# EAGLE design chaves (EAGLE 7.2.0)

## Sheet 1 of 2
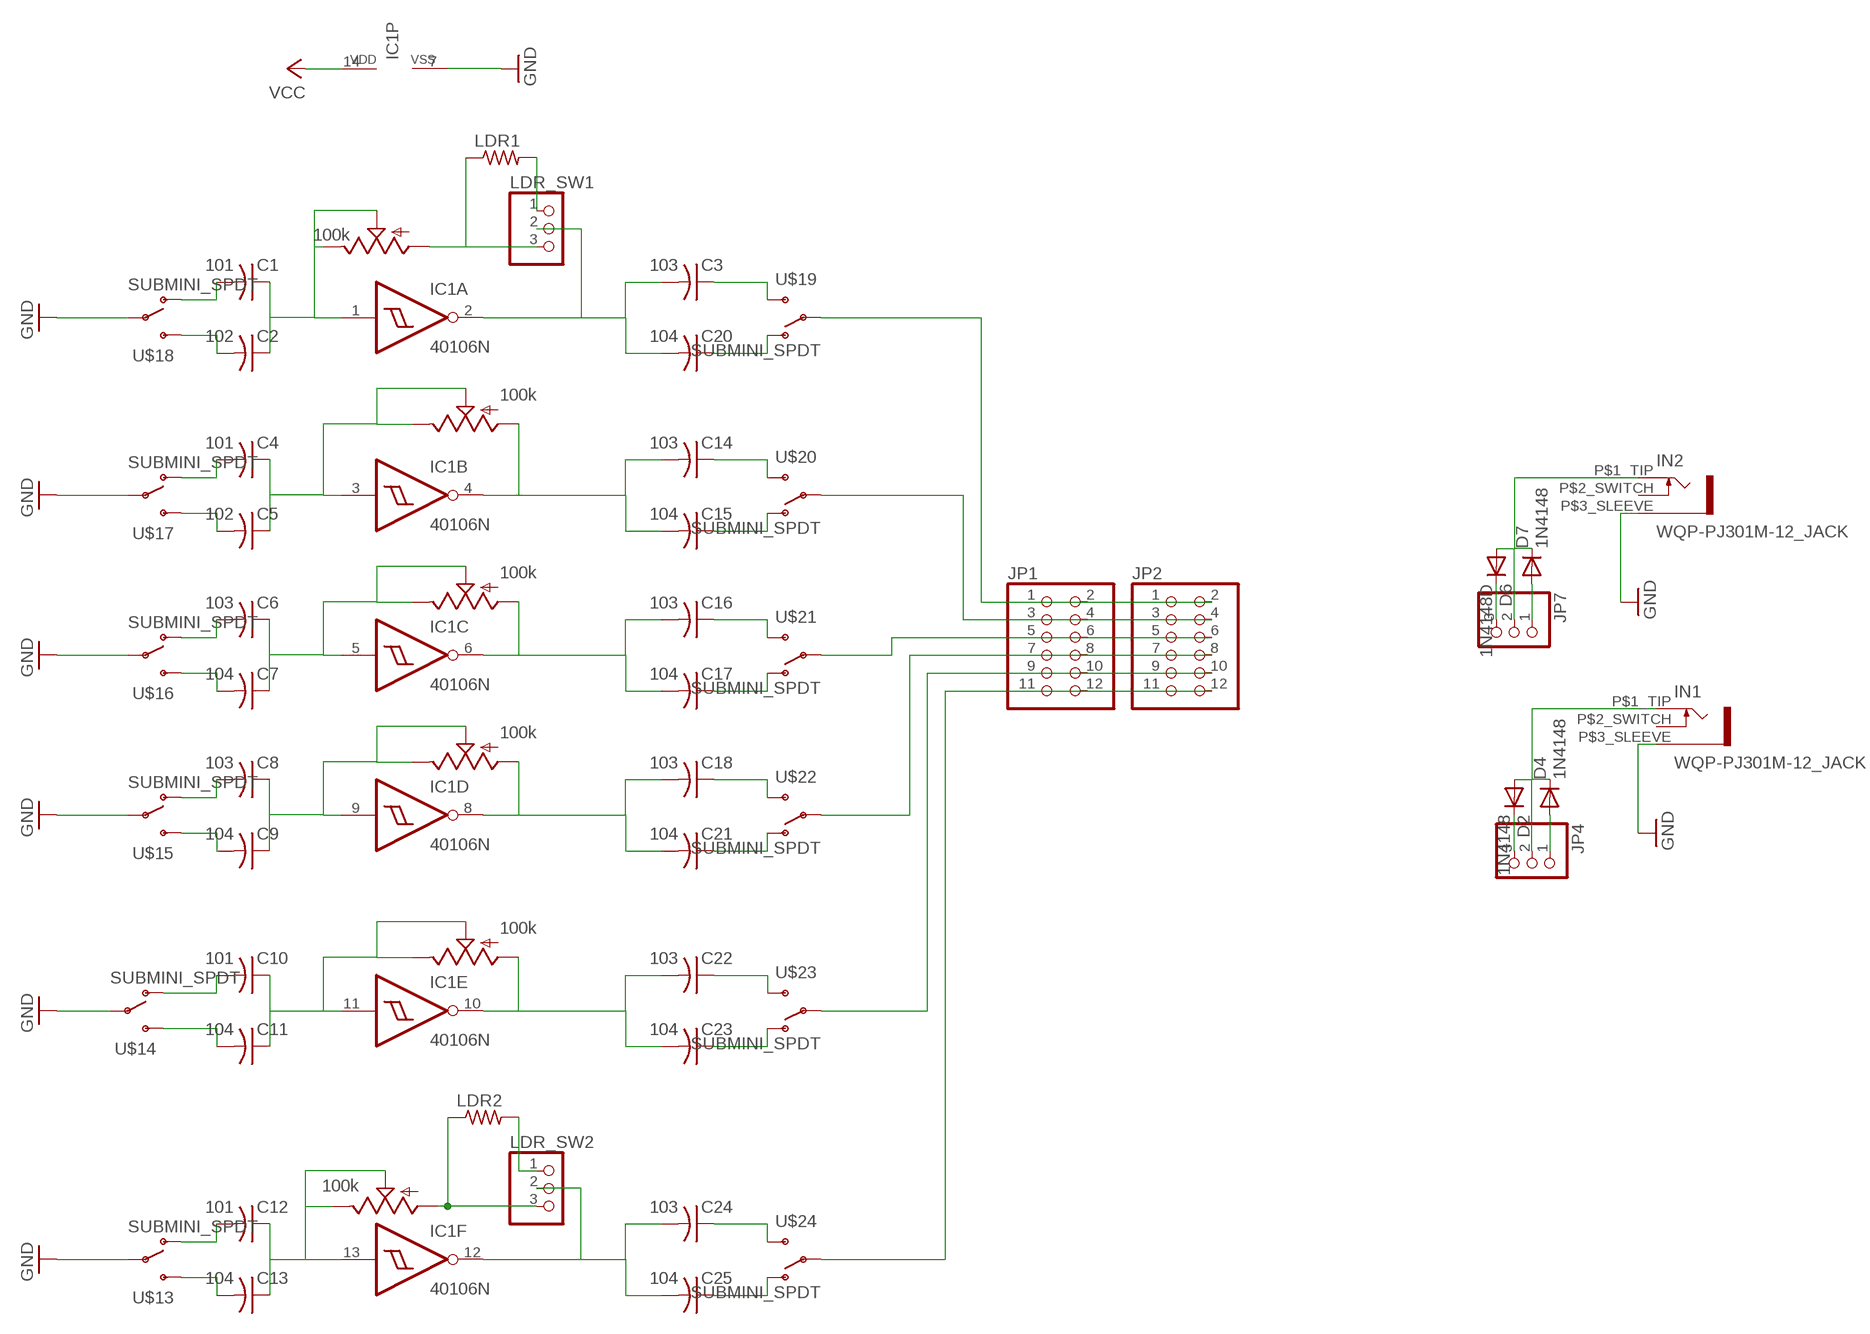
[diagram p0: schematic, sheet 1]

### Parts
C1  101  C-US050-025X075  [C050-025X075]
C2  102  C-US050-025X075  [C050-025X075]
C3  103  C-US050-025X075  [C050-025X075]
C4  101  C-US050-025X075  [C050-025X075]
C5  102  C-US050-025X075  [C050-025X075]
C6  103  C-US050-025X075  [C050-025X075]
C7  104  C-US050-025X075  [C050-025X075]
C8  103  C-US050-025X075  [C050-025X075]
C9  104  C-US050-025X075  [C050-025X075]
C10  101  C-US050-025X075  [C050-025X075]
C11  104  C-US050-025X075  [C050-025X075]
C12  101  C-US050-025X075  [C050-025X075]
C13  104  C-US050-025X075  [C050-025X075]
C14  103  C-US050-025X075  [C050-025X075]
C15  104  C-US050-025X075  [C050-025X075]
C16  103  C-US050-025X075  [C050-025X075]
C17  104  C-US050-025X075  [C050-025X075]
C18  103  C-US050-025X075  [C050-025X075]
C20  104  C-US050-025X075  [C050-025X075]
C21  104  C-US050-025X075  [C050-025X075]
C22  103  C-US050-025X075  [C050-025X075]
C23  104  C-US050-025X075  [C050-025X075]
C24  103  C-US050-025X075  [C050-025X075]
C25  104  C-US050-025X075  [C050-025X075]
D2  1N4148  1N4148DO35-7  [DO35-7]
D4  1N4148  1N4148DO35-7  [DO35-7]
D6  1N4148D  1N4148DO35-7  [DO35-7]
D7  1N4148  1N4148DO35-7  [DO35-7]
IC1  40106N  [DIL14]
IN1  WQP-PJ301M-12_JACK  [WQP-PJ301M-12_JACK]
IN2  WQP-PJ301M-12_JACK  [WQP-PJ301M-12_JACK]
JP1  PINHD-2X6  [2X06]
JP2  PINHD-2X6  [2X06]
JP4  PINHD-1X3CB  [1X03-CLEANBIG]
JP7  PINHD-1X3CB  [1X03-CLEANBIG]
LDR1  R-US_0204/7  [0204/7]
LDR2  R-US_0204/7  [0204/7]
LDR_SW1  PINHD-1X3  [1X03]
LDR_SW2  PINHD-1X3  [1X03]
POT1  100k  POT_USVERTICAL  [ALPS_POT_VERTICAL]
POT2  100k  POT_USVERTICAL  [ALPS_POT_VERTICAL]
POT3  100k  POT_USVERTICAL  [ALPS_POT_VERTICAL]
POT4  100k  POT_USVERTICAL  [ALPS_POT_VERTICAL]
POT5  100k  POT_USVERTICAL  [ALPS_POT_VERTICAL]
POT6  100k  POT_USVERTICAL  [ALPS_POT_VERTICAL]
U$13  SUBMINI_SPDT  [SUBMINI_TOGGLE]
U$14  SUBMINI_SPDT  [SUBMINI_TOGGLE]
U$15  SUBMINI_SPDT  [SUBMINI_TOGGLE]
U$16  SUBMINI_SPDT  [SUBMINI_TOGGLE]
U$17  SUBMINI_SPDT  [SUBMINI_TOGGLE]
U$18  SUBMINI_SPDT  [SUBMINI_TOGGLE]
U$19  SUBMINI_SPDT  [SUBMINI_TOGGLE]
U$20  SUBMINI_SPDT  [SUBMINI_TOGGLE]
U$21  SUBMINI_SPDT  [SUBMINI_TOGGLE]
U$22  SUBMINI_SPDT  [SUBMINI_TOGGLE]
U$23  SUBMINI_SPDT  [SUBMINI_TOGGLE]
U$24  SUBMINI_SPDT  [SUBMINI_TOGGLE]

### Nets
GND: IC1.7(P:VSS) IN1.P$3_SLEEVE IN2.P$3_SLEEVE U$13.COM(COMMON) U$14.COM(COMMON) U$15.COM(COMMON) U$16.COM(COMMON) U$17.COM(COMMON) U$18.COM(COMMON) ; also sheet 2
GND1: C3.2 C20.2 IC1.2(A:O) LDR_SW1.2
GND2: C14.2 C15.2 IC1.4(B:O) POT2.P$3(A)
GND3: C16.2 C17.2 IC1.6(C:O) POT3.P$3(A)
GND4: C18.2 C21.2 IC1.8(D:O) POT4.P$3(A)
GND5: C22.2 C23.2 IC1.10(E:O) POT5.P$3(A)
GND6: C24.2 C25.2 IC1.12(F:O) LDR_SW2.2
N$1: C1.2 U$18.1(O)
N$2: C2.2 U$18.3(S)
N$3: LDR2.2 LDR_SW2.1
N$4: C5.2 U$17.3(S)
N$5: C4.2 U$17.1(O)
N$6: LDR1.2 LDR_SW1.1
N$7: C8.2 U$15.1(O)
N$8: C9.2 U$15.3(S)
N$9: D6.A D7.C IN2.P$1_TIP JP7.2
N$10: C6.2 U$16.1(O)
N$11: C7.2 U$16.3(S)
N$16: C20.1 U$19.1(O)
N$17: C3.1 U$19.3(S)
N$18: JP1.1 JP1.2 JP2.1 JP2.2 U$19.COM(COMMON)
N$19: LDR1.1 LDR_SW1.3 POT1.P$3(A)
N$22: LDR2.1 LDR_SW2.3 POT6.P$3(A)
N$23: D2.A D4.C IN1.P$1_TIP JP4.2
N$24: C15.1 U$20.1(O)
N$26: C14.1 U$20.3(S)
N$27: JP1.3 JP1.4 JP2.3 JP2.4 U$20.COM(COMMON)
N$28: C17.1 U$21.1(O)
N$29: C16.1 U$21.3(S)
N$30: JP1.5 JP1.6 JP2.5 JP2.6 U$21.COM(COMMON)
N$31: C1.1 C2.1 IC1.1(A:I) POT1.P$1(E) POT1.P$2(S)
N$32: C4.1 C5.1 IC1.3(B:I) POT2.P$1(E) POT2.P$2(S)
N$33: C6.1 C7.1 IC1.5(C:I) POT3.P$1(E) POT3.P$2(S)
N$34: C8.1 C9.1 IC1.9(D:I) POT4.P$1(E) POT4.P$2(S)
N$37: C21.1 U$22.1(O)
N$38: C18.1 U$22.3(S)
N$39: JP1.7 JP1.8 JP2.7 JP2.8 U$22.COM(COMMON)
N$40: C23.1 U$23.1(O)
N$41: C22.1 U$23.3(S)
N$42: JP1.9 JP1.10 JP2.9 JP2.10 U$23.COM(COMMON)
N$43: C25.1 U$24.1(O)
N$44: C24.1 U$24.3(S)
N$45: JP1.11 JP1.12 JP2.11 JP2.12 U$24.COM(COMMON)
N$46: C10.2 U$14.1(O)
N$47: C10.1 C11.1 IC1.11(E:I) POT5.P$1(E) POT5.P$2(S)
N$48: C11.2 U$14.3(S)
N$49: C13.2 U$13.3(S)
N$50: C12.2 U$13.1(O)
N$51: C12.1 C13.1 IC1.13(F:I) POT6.P$1(E) POT6.P$2(S)
N$52: D2.C JP4.3
N$53: D4.A JP4.1
N$56: D6.C JP7.3
N$58: D7.A JP7.1
VCC: IC1.14(P:VDD) ; also sheet 2
Unconnected: IN1.P$2_SWITCH IN2.P$2_SWITCH

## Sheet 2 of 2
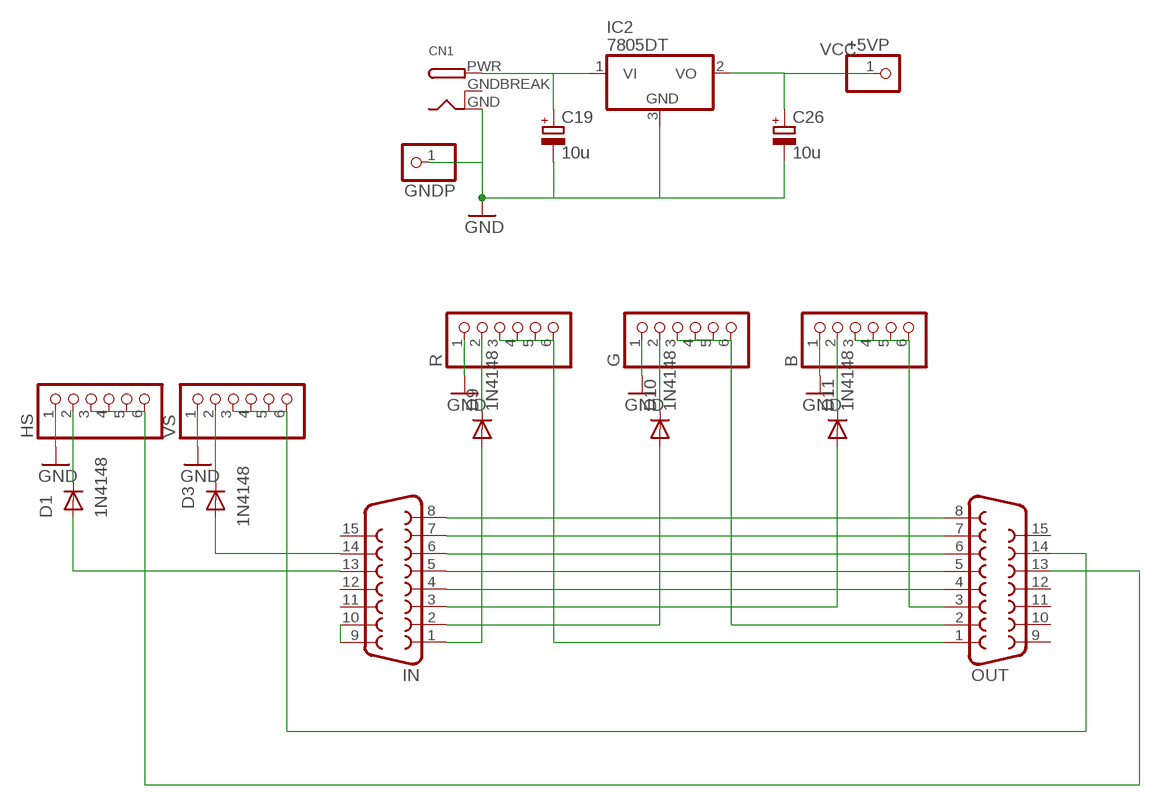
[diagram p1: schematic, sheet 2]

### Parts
+5VP  PINHD-1X1CB  [1X01-CLEANBIG]
B  PINHD-1X6CLEAN  [1X06-CLEAN]
C19  10u  CPOL-EUE2.5-5  [E2,5-5]
C26  10u  CPOL-EUE2.5-5  [E2,5-5]
CN1  DCBARRELPTH  [DCJACK_2MM_PTH]
D1  1N4148  1N4148DO35-7  [DO35-7]
D3  1N4148  1N4148DO35-7  [DO35-7]
D9  1N4148  1N4148DO35-7  [DO35-7]
D10  1N4148  1N4148DO35-7  [DO35-7]
D11  1N4148  1N4148DO35-7  [DO35-7]
G  PINHD-1X6CLEAN  [1X06-CLEAN]
GNDP  PINHD-1X1CB  [1X01-CLEANBIG]
HS  PINHD-1X6CLEAN  [1X06-CLEAN]
IC2  7805DT  [TO252]
IN  F15HDH  [HDF15H]
OUT  F15HDH  [HDF15H]
R  PINHD-1X6CLEAN  [1X06-CLEAN]
VS  PINHD-1X6CLEAN  [1X06-CLEAN]

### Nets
GND: B.1 C19.- C26.- CN1.GND G.1 GNDP.1 HS.1 IC2.3(GND) IN.4 IN.5 IN.6 IN.7 IN.8 IN.9 IN.10 OUT.4 OUT.5 OUT.6 OUT.7 OUT.8 R.1 VS.1 ; also sheet 1
N$12: D9.A IN.1
N$13: D9.C R.2
N$14: OUT.1 R.3 R.4 R.5 R.6
N$15: D10.A IN.2
N$20: D10.C G.2
N$21: G.3 G.4 G.5 G.6 OUT.2
N$25: D11.A IN.3
N$35: B.2 D11.C
N$36: B.3 B.4 B.5 B.6 OUT.3
N$54: OUT.14 VS.3 VS.4 VS.5 VS.6
N$55: HS.3 HS.4 HS.5 HS.6 OUT.13
N$57: C19.+ CN1.PWR IC2.1(VI)
N$60: D1.C HS.2
N$62: D1.A IN.13
N$63: D3.A IN.14
N$64: D3.C VS.2
VCC: +5VP.1 C26.+ IC2.2(VO) ; also sheet 1
Unconnected: IN.11 IN.12 IN.15 OUT.9 OUT.10 OUT.11 OUT.12 OUT.15

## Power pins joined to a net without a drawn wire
GNDBREAK: CN1.GNDBREAK

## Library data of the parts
+5VP GNDP = adafruit:PINHD-1X1: Pin header 1x1 for 0.1" spacing
B G HS R VS = adafruit:PINHD-1X6: PIN HEADER
C1-C18 C20-C25 = adafruit:C-US: CAPACITOR, American symbol
C19 C26 = rcl:CPOL-EU: POLARIZED CAPACITOR, European symbol
CN1 = adafruit:DCBARREL: 2.0mm DC Barrel Jack DCJACK_2MM_PTH - Through Hole Jack (4UConnector: 05537)
D1-D4 D6 D7 D9-D11 = diode:1N4148: DIODE
IC1 = 40xx:40106: Hex SCHMITT TRIGGER
IC2 = adafruit:78*: Positive VOLTAGE REGULATOR Added bigger pads to the TO-92 package
IN OUT = adafruit:F15: SUB-D HDH is also known as a 'right angle VGA' connector
IN1 IN2 = MusicThingModular:WQP-PJ301M-12_JACK
JP1 JP2 = pinhead:PINHD-2X6: PIN HEADER
JP4 JP7 = adafruit:PINHD-1X3: PIN HEADER
LDR1 LDR2 = adafruit:R-US_: RESISTOR, American symbol
LDR_SW1 LDR_SW2 = pinhead:PINHD-1X3: PIN HEADER
POT1-POT6 = pot-alps:POT_US
U$13-U$24 = MusicThingModular:SUBMINI_SPDT

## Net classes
0 default: width 0.406 mm, drill 0.254 mm, clearance 0.254 mm

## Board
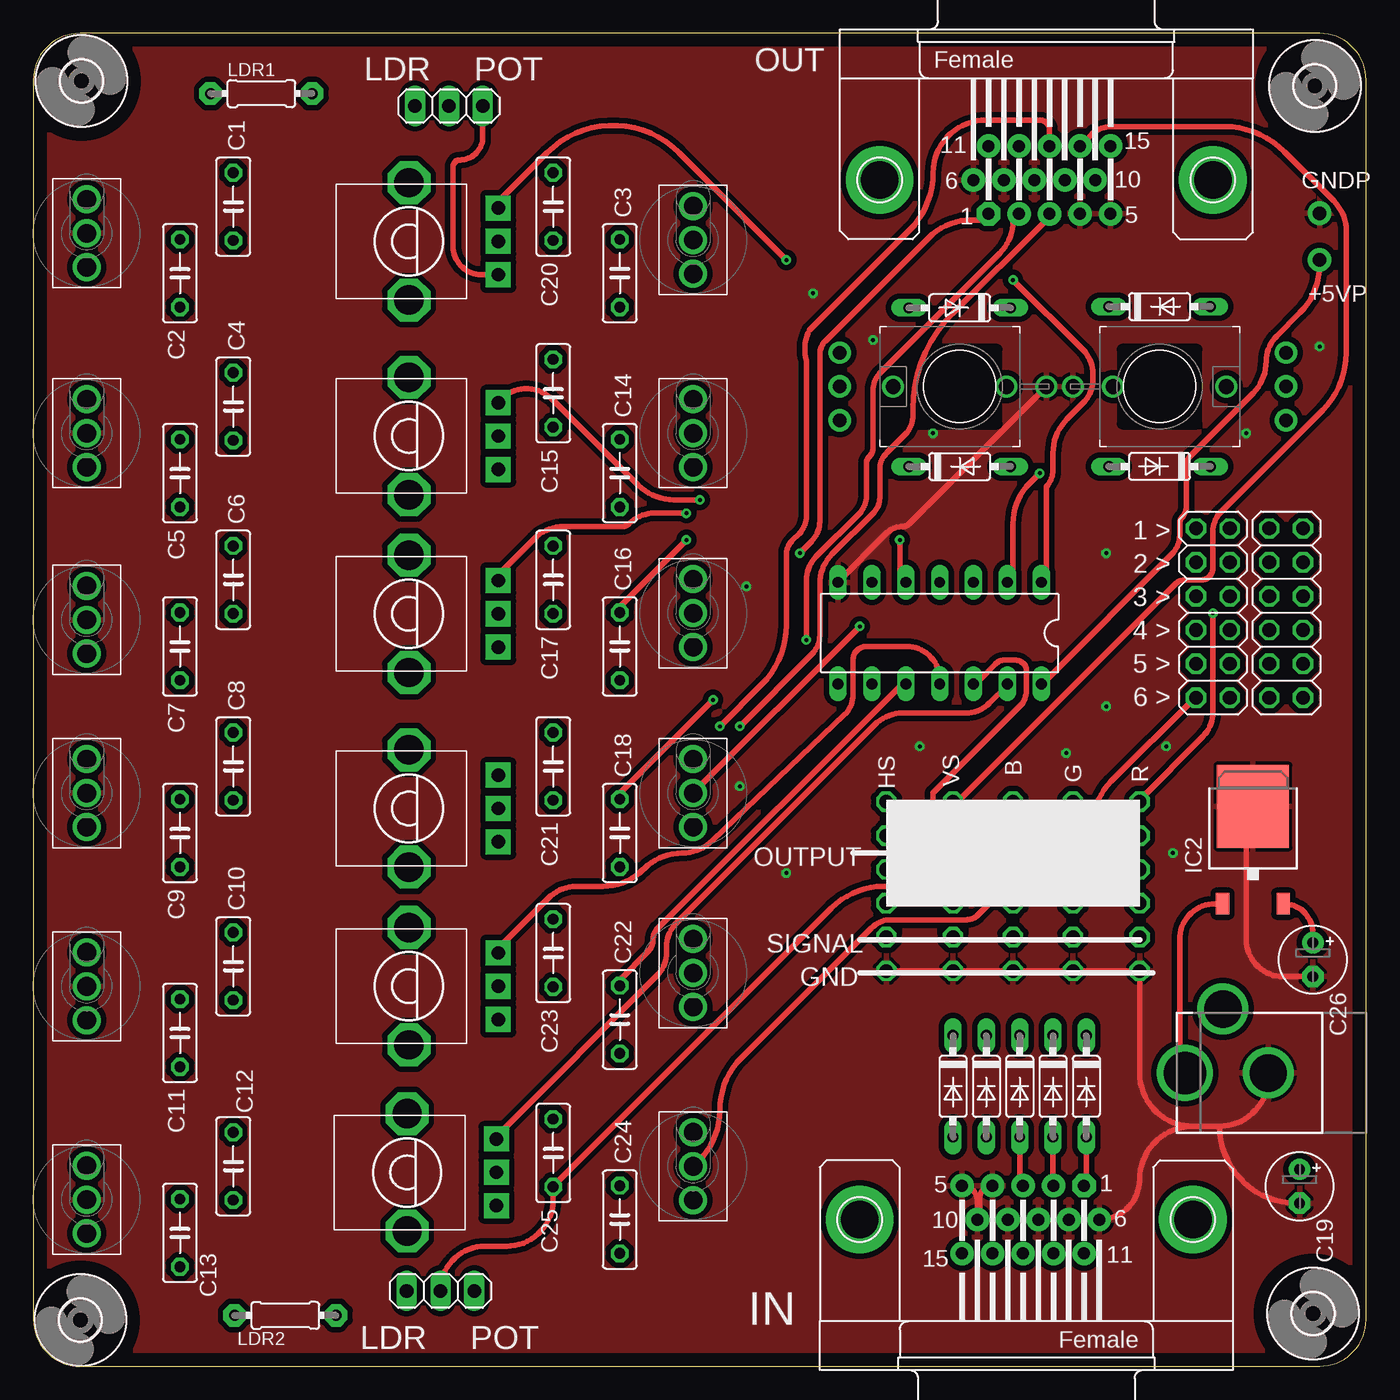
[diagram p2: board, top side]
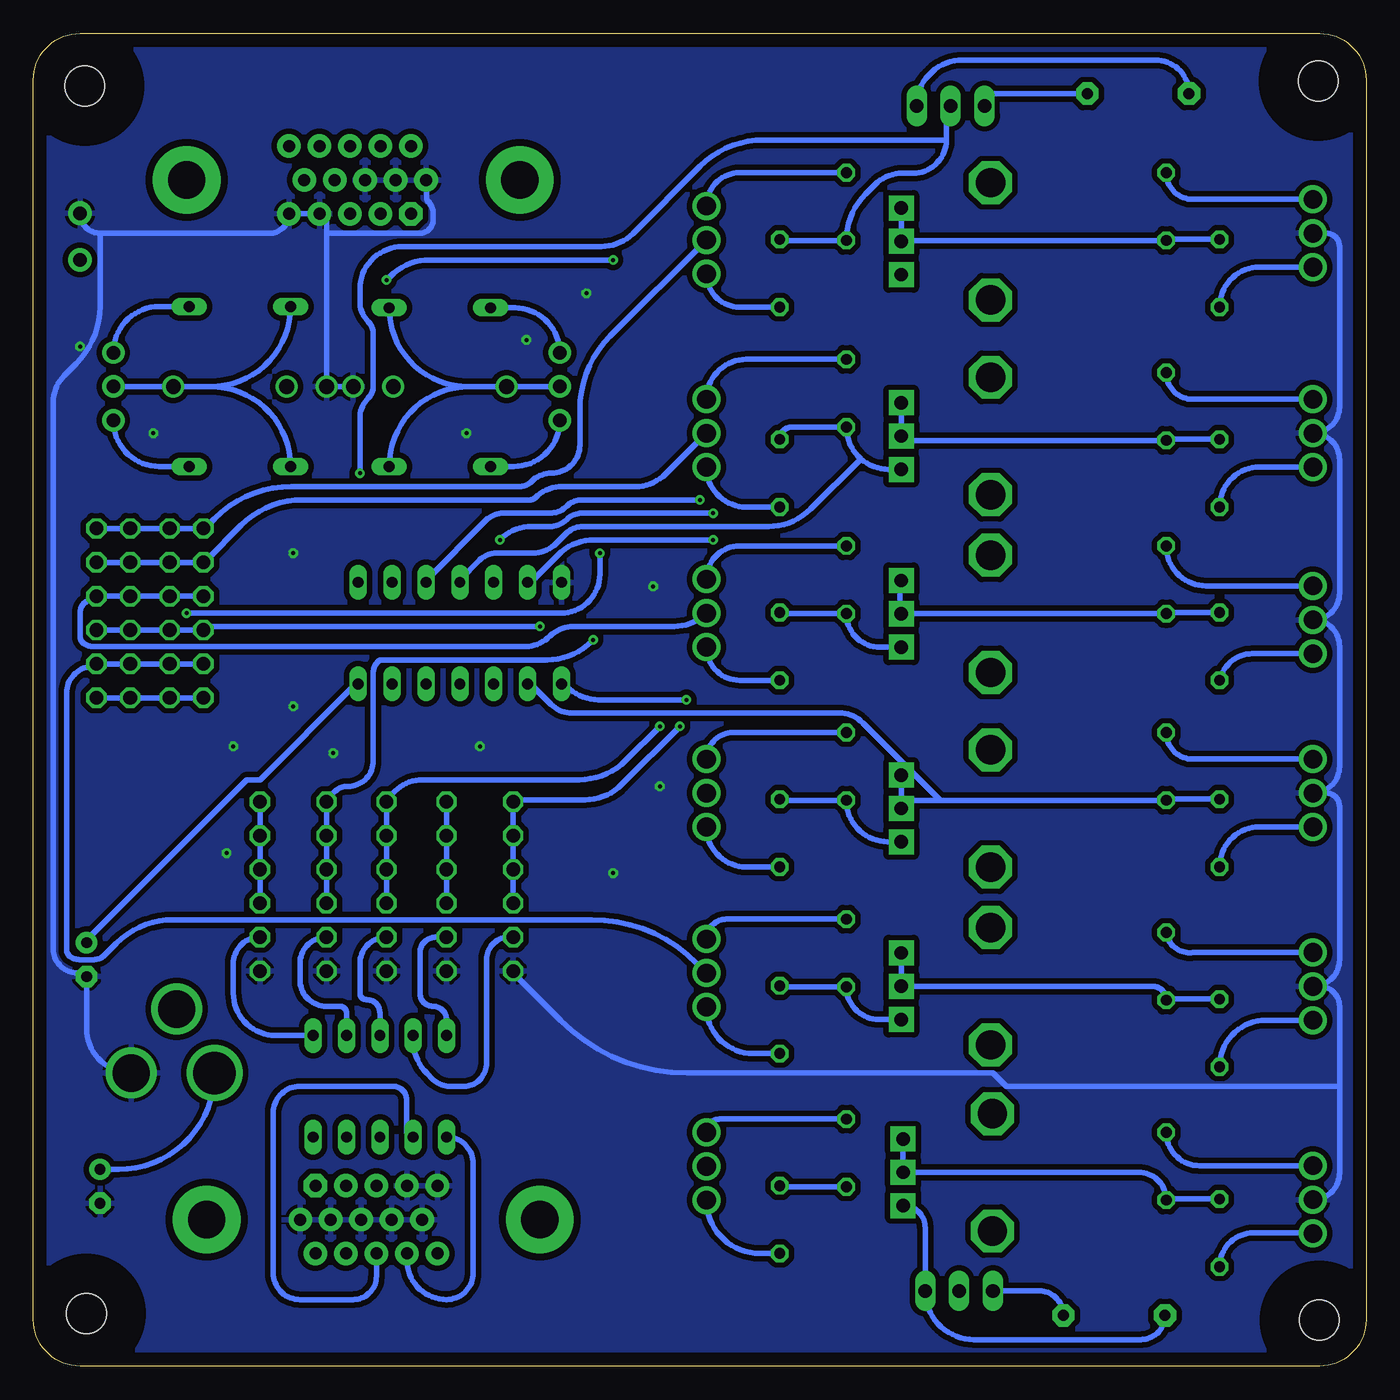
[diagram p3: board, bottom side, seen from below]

Size 100 x 100 mm. Coordinates in mm from the lower left corner, seen from the top.
Outline: 0,96.5 0,3.5 arc90 3.5,0 96.5,0 arc90 100,3.5 100,96.5 arc90 96.5,100 3.5,100 arc90 0,96.5
Copper layers (1*16): Top 0.035mm / dielectric 1.5mm / Bottom 0.035mm
Design rules "default *": minimum track width 10mil, minimum drill 24mil, track to track 8mil, track to pad 8mil, pad to pad 8mil, via to via 8mil, smd to smd 8mil, copper to edge 40mil, drill to drill 8mil, minimum pad ring 10mil, minimum via ring 8mil, stop-mask expansion 4mil, vias tented up to drill 0.33mm, thermal gap 10mil

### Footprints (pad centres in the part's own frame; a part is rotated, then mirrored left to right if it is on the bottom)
1X01-CLEANBIG = drill 1.016 pad 1.778: 1 0,0
1X06-CLEAN = drill 1.016 octagon: 1 -6.35,0; 2 -3.81,0; 3 -1.27,0; 4 1.27,0; 5 3.81,0; 6 6.35,0
C050-025X075 = drill 0.813 octagon: 1 -2.54,0; 2 2.54,0
E2,5-5 = drill 0.813 pad 1.6: + -1.27,0 | drill 0.813 pad 1.6 octagon: - 1.27,0
DCJACK_2MM_PTH = drill 2.8: GND 0,7.35; GNDBREAK 4.8,10.75 | drill 3.2: PWR 0,13.6
DO35-7 = drill 0.813 long: A 3.81,0; C -3.81,0
3,0 = hole 3: 0,0
DIL14 = drill 0.813 long: 1 -7.62,-3.81; 2 -5.08,-3.81; 3 -2.54,-3.81; 4 0,-3.81; 5 2.54,-3.81; 6 5.08,-3.81; 7 7.62,-3.81; 8 7.62,3.81; 9 5.08,3.81; 10 2.54,3.81; 11 0,3.81; 12 -2.54,3.81; 13 -5.08,3.81; 14 -7.62,3.81
TO252 = smd 1 x 1.6: 1 -2.28,-4.8; 2 2.28,-4.8 | smd 5.4 x 6.2: 3 0,2.5
HDF15H = drill 0.9 pad 1.778 octagon: 1 4.329,2.54 | drill 0.9 pad 1.778: 2 2.043,2.54; 3 -0.243,2.54; 4 -2.529,2.54; 5 -4.815,2.54; 6 5.472,0; 7 3.186,0; 8 0.9,0; 9 -1.386,0; 10 -3.672,0; 11 4.329,-2.54; 12 2.043,-2.54; 13 -0.243,-2.54; 14 -2.529,-2.54; 15 -4.815,-2.54 | drill 2.8 pad 5.08: P$1 -12.5,0; P$2 12.5,0
WQP-PJ301M-12_JACK = drill 1.1: P$1_TIP 0,5; P$2_SWITCH 0,-3.5; P$3_SLEEVE 0,-6.5
2X06 = drill 1.016 octagon: 1 -6.35,-1.27; 2 -6.35,1.27; 3 -3.81,-1.27; 4 -3.81,1.27; 5 -1.27,-1.27; 6 -1.27,1.27; 7 1.27,-1.27; 8 1.27,1.27; 9 3.81,-1.27; 10 3.81,1.27; 11 6.35,-1.27; 12 6.35,1.27
1X03-CLEANBIG = drill 1.016 pad 1.676: 1 -2.54,0; 2 0,0; 3 2.54,0
0204/7 = drill 0.813 pad 1.676 octagon: 1 -3.81,0; 2 3.81,0
1X03 = drill 1.016 long: 1 -2.54,0; 2 0,0; 3 2.54,0
ALPS_POT_VERTICAL = drill 1 pad 1.88 square: P$1 -2.5,6.7; P$2 0,6.7; P$3 2.5,6.7 | drill 2.2 pad 3.175 octagon: P$4 -4.4,0; P$5 4.4,0
SUBMINI_TOGGLE = drill 1.4 pad 1.829: 1 -2.54,0; 3 2.54,0; COM 0,0

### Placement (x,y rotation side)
+5VP  96.5,83 0 top
B  73.5,36 90 top
C1  15,87 90 top
C2  11,82 270 top
C3  44,82 90 top
C4  15,72 90 top
C5  11,67 270 top
C6  15,59 90 top
C7  11,54 270 top
C8  15,45 90 top
C9  11,40 270 top
C10  15,30 90 top
C11  11,25 270 top
C12  15,15 90 top
C13  11,10 270 top
C14  44,67 90 top
C15  39,73 270 top
C16  44,54 90 top
C17  39,59 270 top
C18  44,40 90 top
C19  95,13.5 270 top
C20  39,87 270 top
C21  39,45 270 top
C22  44,26 90 top
C23  39,31 270 top
C24  44,11 90 top
C25  39,16 270 top
C26  96,30.5 270 top
CN1  100,22 90 top
D1  71.5,21 270 top
D2  84.5,67.5 180 top
D3  69,21 270 top
D4  84.5,79.5 0 top
D6  69.5,67.5 0 top
D7  69.5,79.4 180 top
D9  79,21 270 top
D10  76.5,21 270 top
D11  74,21 270 top
E$1  [3,0]  96.02,3.95 0 top
E$5  [3,0]  3.52,3.45 0 top
E$7  [3,0]  3.6,96.42 0 top
E$8  [3,0]  96.15,96.06 0 top
G  78,36 90 top
GNDP  96.5,86.5 0 top
HS  64,36 90 top
IC1  68,55 180 top
IC2  91.5,39.5 0 top
IN  74.5,11 0 top
IN1  84.5,73.5 270 top
IN2  69.5,73.5 90 top
JP1  88.5,56.5 270 top
JP2  94,56.5 270 top
JP4  94,73.5 270 top
JP7  60.5,73.5 270 top
LDR1  17.11,95.48 0 top
LDR2  18.91,3.81 0 top
LDR_SW1  31.18,94.55 0 top
LDR_SW2  30.55,5.65 0 top
OUT  76,89 180 top
POT1  28.18,84.39 270 top
POT2  28.18,69.78 270 top
POT3  28.18,56.45 270 top
POT4  28.18,41.84 270 top
POT5  28.18,28.51 270 top
POT6  28.05,14.54 270 top
R  83,36 90 top
U$13  4,12.5 270 top
U$14  4,28.5 270 top
U$15  4,43 270 top
U$16  4,56 270 top
U$17  4,70 270 top
U$18  4,85 270 top
U$19  49.5,84.5 270 top
U$20  49.5,70 270 top
U$21  49.5,56.5 270 top
U$22  49.5,43 270 top
U$23  49.5,29.5 270 top
U$24  49.5,15 270 top
VS  69,36 90 top

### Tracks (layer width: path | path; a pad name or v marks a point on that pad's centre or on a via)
GND  (via drill 0.3)
  Top 0.406: CN1.GND 92.65,21.65 arc-90 89,18 | 89,18 87,18 | 87,18 arc-90 83,22 R.1 G.1 B.1 VS.1 HS.1 | IN.5 arc-90 70.83,12.4 IN.10 71,11 | 71,11 71,12.57 arc-90 IN.4 | 71,11 IN.9 IN.8 IN.7 IN.6 80,11 arc90 83,14 arc-90 87,18 | C19.- 94.77,12.23 arc-90 89,18 | C26.- 93.77,29.23 arc-90 91,32 91,41 arc-90 92,42 IC2.3 | OUT.6 OUT.7 OUT.8 | IN2.P$3_SLEEVE 65.68,63.18 arc-45 65.25,63 arc45 63.97,62.47 60.5,59 IC1.7
  Bottom 0.406: U$13.COM arc-90 2,14.5 2,21 | 2,21 2,27 arc-90 3.5,28.5 U$14.COM arc-90 2,30.5 2,42 arc-90 3,43 U$15.COM arc-90 2,45 2,54 arc-90 U$16.COM arc-90 2,58 2,68 arc-90 U$17.COM arc-90 2,72 2,84 arc-90 3,85 U$18.COM | CN1.GND arc90 96,25.35 C26.- 96,29.5 96.7,29.5 arc90 98.5,31.3 98.5,72.33 arc45 97.67,74.33 96.77,75.23 arc-45 95,79.5 95,85 | IN2.P$3_SLEEVE IN1.P$3_SLEEVE 78,85 | 78,85 78,85.93 arc-90 OUT.4 OUT.5 arc90 82.28,85 95,85 | 95,85 arc90 GNDP.1 | 78,85 71,85 arc-90 70,86 70,86.5 arc-45 70.35,87.35 arc45 70.5,87.71 70.5,89 OUT.6 | 2,21 27,21 28,22 50.94,22 arc45 60.44,25.93 64,29.5 HS.1
  other vias: 56.5,37 53,43.5 58.5,80.5 66.5,46.5 85,46.5 63,77 91,70 80.5,49.5 96.5,76.5 53.5,58.5 80.5,61 77.5,46 85.5,38.5 67.5,70
  pour Top (isolate 0.406): 0,100 100,100 100,0 0,0
  pour Bottom (isolate 0.406): 0,100 100,100 100,0 0,0
GND1  (via drill 0.3)
  Top 0.406: v75.5,67 74.75,66.25 arc45 73.5,63.23 73.5,59 IC1.2
  Bottom 0.406: C3.2 arc-90 43.92,84.46 C20.2 arc45 37.56,87.94 36.85,88.65 arc45 34.79,89.5 34,89.5 arc-90 31.5,92 | LDR_SW1.2 arc-90 31.5,94.23 31.5,92 | v75.5,67 75.5,71.12 arc45 74.88,72.62 arc-45 74.5,73.54 74.5,77.46 arc-45 74.88,78.38 arc45 75.5,79.88 75.5,80.8 arc90 72.3,84 57.39,84 arc-45 55.02,84.98 49.97,90.03 arc45 45.21,92 31.5,92
GND2
  Bottom 0.406: C14.2 arc90 43.08,70.46 C15.2 arc-49 37.93,68.08 | POT2.P$3 35.83,67.28 arc41 37.93,68.08 | IC1.4 68,59 66.53,60.47 arc45 65.25,61 62.54,61 arc-45 60.77,61.73 60.03,62.47 arc45 58.75,63 44.85,63 arc-45 41.69,64.31 38,68 37.93,68.08
GND3  (via drill 0.3)
  Top 0.406: v49,62 44,57 C16.2
  Bottom 0.406: POT3.P$3 36.49,53.95 arc90 C17.2 43.92,56.46 arc90 C16.2 | v49,62 57.88,62 arc-45 60.64,60.86 62.5,59 IC1.6
GND4  (via drill 0.3)
  Top 0.406: v51,50 44,43 C18.2
  Bottom 0.406: POT4.P$3 35.88,39.34 arc90 C21.2 43.92,42.46 arc90 C18.2 | v51,50 57.59,50 arc45 60,51 IC1.8
GND5
  Top 0.406: IC1.10 65,51 46.83,32.83 arc45 46.5,32.04 arc-45 46.12,31.12 44,29 C22.2
  Bottom 0.406: POT5.P$3 36.55,26.01 arc90 C23.2 43.92,28.46 arc90 C22.2
GND6
  Top 0.406: LDR_SW2.2 arc-90 33.9,9 35.5,9 arc90 39,12.5 C25.2 39,13.5 59.88,34.38 arc-45 63.79,36 64.5,36 67.5,39 67.5,43 74.06,49.56 arc45 74.5,50.62 74.5,52.26 arc45 74.33,52.67 arc45 73.54,53 72.96,53 arc45 72.17,52.67 71,51.5 IC1.12
  Bottom 0.406: C25.2 43.92,13.46 arc90 C24.2
N$1
  Bottom 0.406: U$18.1 13,87.54 arc90 C1.2
N$2
  Bottom 0.406: U$18.3 8,82.46 arc-90 C2.2
N$3
  Bottom 0.406: LDR2.2 arc-90 24.55,5.65 LDR_SW2.1
N$4
  Bottom 0.406: U$17.3 8,67.46 arc-90 C5.2
N$5
  Bottom 0.406: U$17.1 13,72.54 arc90 C4.2
N$6
  Bottom 0.406: LDR1.2 27.71,95.48 arc-90 LDR_SW1.1
N$7
  Bottom 0.406: U$15.1 13,45.54 arc90 C8.2
N$8
  Bottom 0.406: U$15.3 8,40.46 arc-90 C9.2
N$9
  Bottom 0.406: JP7.2 IN2.P$1_TIP 67.31,73.5 | 67.31,73.5 67.41,73.5 arc90 D7.C | D6.A arc90 67.31,73.5
N$10
  Bottom 0.406: U$16.1 12,58.54 arc90 C6.2
N$11
  Bottom 0.406: U$16.3 8.54,53.46 arc-90 11,51 C7.2
N$12
  Top 0.406: D9.A 79,13.71 arc-90 IN.1
N$13
  Bottom 0.406: D9.C 81.81,24.81 arc90 85,28 85,30.19 arc90 R.2
N$14  (via drill 0.3)
  Top 0.406: v57.5,61 58.38,61.88 arc45 59,63.38 59,75.91 arc-45 59.41,76.91 67.15,84.65 arc-45 70.41,86 71.5,86 OUT.1 | v88.5,56.5 88.5,49.06 arc-45 87.75,47.25 83,42.5 R.6
  Bottom 0.406: R.6 R.5 | R.5 83,39 | R.5 R.4 R.3 | v88.5,56.5 60.41,56.5 arc-90 57.5,59.41 v57.5,61
N$15
  Top 0.406: D10.A 76.5,13.58 arc90 IN.2
N$16
  Bottom 0.406: C20.1 47,89.54 arc-90 U$19.1
N$17
  Bottom 0.406: C3.1 47,79.46 arc90 U$19.3
N$18
  Bottom 0.406: JP2.2 JP2.1 JP1.2 JP1.1 87,63 86.4,63.6 arc45 80.6,66 63.54,66 arc-45 62.62,66.38 arc45 61.12,67 arc-90 59,69.12 59,71.78 arc45 56.72,77.28 U$19.COM
N$19
  Top 0.406: LDR_SW1.3 33.72,92.22 arc-90 32,90.5 arc90 31.5,90 31.5,84 arc90 33.61,81.89 POT1.P$3
  Bottom 0.406: LDR1.1 arc-90 15.81,98 30.27,98 arc-90 LDR_SW1.3
N$20
  Bottom 0.406: D10.C 76.5,26.5 arc-90 77,27 78,27 arc90 80,29 80,30.19 arc90 G.2
N$21  (via drill 0.3)
  Top 0.406: v58,54.5 58,58.96 arc-45 58.73,60.73 61.97,63.97 arc45 62.5,65.25 62.5,67.71 arc-45 62.71,68.21 arc45 63,68.91 63,73.17 arc-45 63.59,74.59 72.52,83.52 arc45 73.5,85.89 73.5,86 OUT.2
  Bottom 0.406: G.3 G.4 G.5 G.6 78,42.5 77.41,43.09 arc45 76.41,43.5 arc-90 74.5,45.41 74.5,52 arc45 74.15,52.85 arc45 73.79,53 61.45,53 arc-45 58.12,54.38 v58,54.5
N$22
  Bottom 0.406: LDR2.1 arc90 16.91,2 29.43,2 arc90 LDR_SW2.3 33.09,10.38 arc-90 POT6.P$3
N$23
  Bottom 0.406: JP4.2 IN1.P$1_TIP 86.69,73.5 | D2.A arc-90 86.69,73.5 | D4.C arc90 86.69,73.5
N$24
  Bottom 0.406: C15.1 46.5,75.54 arc-90 U$20.1
N$25
  Top 0.406: D11.A 74,13.8 arc90 IN.3
N$26
  Bottom 0.406: C14.1 46.5,64.46 arc90 U$20.3
N$27
  Bottom 0.406: JP2.4 JP2.3 JP1.4 JP1.3 87,60.5 84.41,63.09 arc45 79.8,65 62.71,65 arc-45 62.35,65.15 arc45 60.29,66 54.83,66 arc-45 52.56,66.94 U$20.COM
N$28
  Bottom 0.406: C17.1 47,61.54 arc-90 U$21.1
N$29
  Bottom 0.406: C16.1 47,51.46 arc90 U$21.3
N$30
  Bottom 0.406: JP1.5 JP1.6 JP2.5 JP2.6 95.5,57.5 arc-90 96.5,56.5 96.5,54.79 arc-45 96.29,54.29 arc-45 95.59,54 63.09,54 arc-45 61.23,54.77 arc45 59.46,55.5 51.91,55.5 arc-45 U$21.COM
N$31  (via drill 0.3)
  Top 0.406: v73.5,81.5 78.77,76.23 arc-45 79.5,74.46 79.5,74.06 arc-45 78.75,72.25 77.56,71.06 arc45 76.5,68.51 76.5,67.21 arc-45 76,66 76,59 IC1.1 | v56.5,83 48.46,91.04 arc90 38.54,91.04 34.5,87 POT1.P$1
  Bottom 0.406: C2.1 14.92,84.54 arc-90 C1.1 34.81,84.46 arc-90 POT1.P$2 POT1.P$1 | v56.5,83 70.24,83 arc-45 73.24,81.76 v73.5,81.5
N$32  (via drill 0.3)
  Top 0.406: v50,65 48.08,65 arc-45 45.38,66.11 39,72.5 arc90 35,72.5 POT2.P$1
  Bottom 0.406: C5.1 14.92,69.54 arc-90 C4.1 34.55,69.46 arc90 POT2.P$2 POT2.P$1 | v50,65 58.83,65 arc-45 59.97,64.53 arc45 61.25,64 64.75,64 arc-45 66.03,63.47 70.5,59 IC1.3
N$33  (via drill 0.3)
  Top 0.406: v65,62 65,59 IC1.5 | v49,64 46.62,64 arc45 44.71,63.21 arc-45 44.2,63 39.83,63 arc45 37.56,62.06 34.5,59 POT3.P$1
  Bottom 0.406: C7.1 14.46,56.54 arc-90 15,56 C6.1 POT3.P$2 arc-90 POT3.P$2 34.88,56.12 arc90 35,56 35,58.83 arc90 POT3.P$1 | v65,62 arc45 62.59,63 61.25,63 arc-45 59.97,63.53 arc45 58.83,64 v49,64
N$34
  Bottom 0.406: C9.1 14.92,42.54 arc-90 C8.1 32,42.46 | 32,42.46 34.27,42.46 arc-90 POT4.P$2 POT4.P$1 | IC1.9 62.5,51 61.16,49.66 arc-45 59.57,49 39.54,49 arc45 37.77,48.27 32,42.5 32,42.46
N$35
  Bottom 0.406: D11.C 74,26.5 arc-90 75,27.5 arc90 75.5,28 75.5,30.19 arc90 B.2
N$36  (via drill 0.3)
  Top 0.406: v53,48 58.41,53.41 arc45 59,54.83 59,58.69 arc-45 59.93,60.93 63.06,64.06 arc45 63.5,65.12 63.5,67.25 arc-45 64.03,68.53 65.41,69.91 arc45 66,71.33 66,71.81 arc-45 68.97,78.97 76,86 OUT.3
  Bottom 0.406: B.3 B.4 B.5 B.6 73.5,42.5 72.85,43.15 arc45 70.79,44 59.05,44 arc-45 55.55,45.45 v53,48
N$37
  Bottom 0.406: C21.1 47.5,47.54 arc-90 U$22.1
N$38
  Bottom 0.406: C18.1 46.5,37.46 arc90 U$22.3
N$39  (via drill 0.3)
  Top 0.406: v62,55.5 U$22.COM
  Bottom 0.406: JP2.8 JP2.7 JP1.8 JP1.7 87,55.5 v62,55.5
N$40
  Bottom 0.406: C23.1 48,33.54 arc-90 U$23.1
N$41
  Bottom 0.406: C22.1 46,23.46 arc90 U$23.3
N$42
  Bottom 0.406: JP1.9 JP1.10 JP2.9 JP2.10 95.5,52.5 arc-90 97.5,50.5 97.5,31.24 arc-45 97.33,30.83 arc-45 96.54,30.5 95.46,30.5 arc-45 94.67,30.83 93.77,31.73 arc45 89.5,33.5 58.13,33.5 arc45 50.23,30.23 U$23.COM
N$43
  Bottom 0.406: C25.1 48.5,18.54 arc-90 U$24.1
N$44
  Bottom 0.406: C24.1 45.5,8.46 arc90 U$24.3
N$45
  Top 0.406: U$24.COM 49.95,15.46 arc45 51.5,19.18 arc-45 53.14,23.14 62.88,32.88 arc-45 64.38,33.5 70.04,33.5 arc45 70.83,33.83 72.71,35.71 arc-45 73.41,36 73.94,36 arc45 75.75,36.75 77.09,38.09 arc-45 78.09,38.5 arc45 78.79,38.79 arc45 79.5,40.5 79.5,40.59 arc-45 80.85,43.85 87,50 JP1.11
  Bottom 0.406: JP2.12 JP2.11 JP1.12 JP1.11
N$46
  Bottom 0.406: U$14.1 13,31.04 arc90 C10.2
N$47
  Top 0.406: POT5.P$1 35,31.5 38.61,35.11 arc-45 40.76,36 42.72,36 arc45 45.76,37.26 45.82,37.32 arc-45 48.67,38.5 arc45 50.94,39.44 60.86,48.89 arc46 61.5,50.38 61.5,53 arc-90 62.5,54 65.5,54 arc-90 68,51.5 IC1.11
  Bottom 0.406: C11.1 14.92,27.54 arc-90 C10.1 arc-90 16.05,28.51 POT5.P$2 | 34.37,28 arc90 POT5.P$2 | POT5.P$2 POT5.P$1
N$48
  Bottom 0.406: U$14.3 7.5,25.96 arc-90 C11.2
N$49
  Bottom 0.406: U$13.3 4,10 8.46,10 arc-90 C13.2
N$50
  Bottom 0.406: U$13.1 12.5,15.04 arc90 C12.2
N$51
  Top 0.406: IC1.13 73,51 71.75,49.75 arc-45 69.94,49 65.26,49 arc45 63.11,48.11 48.23,33.23 arc45 47.5,31.46 47.5,31.04 arc-45 46.77,29.27 35,17.5 POT6.P$1
  Bottom 0.406: C13.1 14.92,12.54 arc-90 C12.1 arc-90 17.08,14.54 POT6.P$2 POT6.P$1
N$52
  Bottom 0.406: D2.C 90.54,67.5 arc90 JP4.3
N$53
  Bottom 0.406: D4.A 90.54,79.5 arc-90 JP4.1
N$54
  Top 0.406: OUT.14 79,92 79.41,92.41 arc-45 80.83,93 89.36,93 arc-45 93.86,91.14 97.56,87.44 arc-45 98.5,85.17 98.5,75.99 arc-45 96.74,71.74 89.12,64.12 arc45 88.5,62.62 88.5,59.91 arc-45 88.21,59.21 arc-45 87.71,59 86.46,59 arc45 85.67,58.67 69,42 VS.6
  Bottom 0.406: VS.3 VS.4 VS.5 VS.6
N$55  (via drill 0.3)
  Top 0.406: v51.5,48 54.66,51.16 arc45 56.5,55.59 56.5,60.84 arc-45 56.96,61.96 57.47,62.47 arc45 58,63.75 58,75.44 arc-45 58.25,77.75 65.73,85.23 arc45 67.5,89.5 arc-90 71.5,93.5 75.5,93.5 arc-90 76.24,92.76 OUT.13
  Bottom 0.406: HS.3 HS.4 HS.5 HS.6 64,42.5 58.62,42.5 arc-45 55.86,43.64 v51.5,48
N$56
  Bottom 0.406: JP7.3 arc90 63.96,67.5 D6.C
N$57
  Top 0.406: IC2.1 88.7,34.7 arc90 86,32 86,22.4 arc90 CN1.PWR
  Bottom 0.406: C19.+ 93.63,14.77 arc-90 CN1.PWR
N$58
  Bottom 0.406: JP7.1 arc-90 63.86,79.4 D7.A
N$60
  Bottom 0.406: D1.C 71.5,24.46 arc-45 70.46,21.96 70.03,21.53 arc-45 68.75,21 67.67,21 arc-45 66.53,21.47 arc-45 66,22.75 66,30.5 arc90 64.31,32.19 HS.2
N$62
  Bottom 0.406: IN.13 74.26,6.74 arc90 76,5 80,5 arc90 82,7 82,19 arc90 80,21 73,21 arc90 72,20 72,17.69 arc-90 D1.A
N$63
  Bottom 0.406: D3.A arc90 67,15.19 67,7 arc90 69,5 arc90 71.97,7.97 IN.14
N$64
  Bottom 0.406: D3.C 69,26 arc-90 70,27 arc90 71,28 71,31 arc90 69.81,32.19 VS.2
VCC
  Top 0.406: C26.+ 96,32.48 arc90 IC2.2 | +5VP.1 96.5,82.58 arc-45 95.03,79.03 93.28,77.28 arc45 92.5,75.39 arc-45 91.52,73.02 86.83,68.33 arc45 86.5,67.54 86.5,64.41 arc-45 86.21,63.71 arc45 86,63.21 86,62.33 arc-45 85.41,60.91 76,51.5 IC1.14
  Bottom 0.406: IC1.14 76,51 83,44 84,44 96,32 C26.+

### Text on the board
tNames: LDR | POT | 1 > | 2 > | 3 > | 4 > | 5 > | 6 > | OUTPUT | SIGNAL | GND | LDR | POT
bValues: CHA/VES - based on jonasbers.com/chav/ | http://github.com/ttreintaysiete/chaves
